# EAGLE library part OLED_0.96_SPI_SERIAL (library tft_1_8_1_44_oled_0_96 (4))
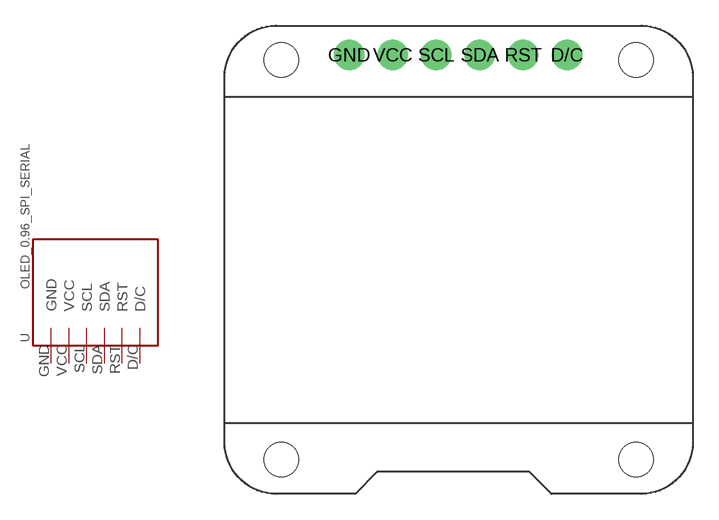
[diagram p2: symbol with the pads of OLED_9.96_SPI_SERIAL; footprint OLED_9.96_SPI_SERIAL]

Designator prefix -

## OLED_0.96_SPI_SERIAL  [OLED_9.96_SPI_SERIAL]
D/C  D/C
GND  GND
RST  RST
SCL  SCL
SDA  SDA
VCC  VCC

## Footprint OLED_9.96_SPI_SERIAL (pad centres in mm)
drill 1 pad 1.778: D/C 5.99,11.63; GND -6.71,11.63; RST 3.45,11.63; SCL -1.63,11.63; SDA 0.91,11.63; VCC -4.17,11.63
hole 2 at -10.67,-11.97
hole 2 at 10.03,-11.97
hole 2 at 10.03,11.33
hole 2 at -10.67,11.33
